PROGRAM MAIN
VAR
	{attribute 'pytmc' := 'pv: PREFIX:fbTest'}
	fbTest : FB_SampleA_Test;
	{attribute 'pytmc' := 'pv: PREFIX:fOutput'}
	fOutput : LREAL;
END_VAR

fbTest(fInput:=1.0, fOutput=>fOutput);

END_PROGRAM
